// TwinCAT 3 PLC project DynTcComProxy
// ProgramVersion: 3.1.4024.0
// libraries:
//   Tc2_Standard, * (Beckhoff Automation GmbH)
//   Tc2_System, * (Beckhoff Automation GmbH)
//   Tc2_Utilities, * (Beckhoff Automation GmbH)
//   Tc3_Module, * (Beckhoff Automation GmbH)
//   TcComProxyApplication, * (YuYang_Beckhoffsh)
// project tree:
//   / PlcTask.TcTTO
//   POUs/ FB_DynProxyTcComConvertModule.TcPOU, MAIN.TcPOU
// real-time tasks:
//   TASK PlcTask: cycle T#10ms, priority 20, ADS port 350
//   TASK PlcTask1: cycle T#10ms, priority 21, ADS port 351
//   TASK PlcTask2: cycle T#10ms, priority 22, ADS port 352
//   TASK PlcTask3: cycle T#10ms, priority 23, ADS port 353
// variable links:
//   TcComPLCCaller/TcComPLCCaller Instance <-> TcComPLCProvider/TcComPLCProvider Instance
//     PlcTask Inputs/MAIN.fbProxyPLCCalculationTcComModule._objectId <-> PlcTask Outputs/MAIN.fbCalc.objID

CONFIGURATION DynTcComProxy
    RESOURCE PLC ON TwinCAT3
        TASK PlcTask(INTERVAL := T#10ms, PRIORITY := 20);
        PROGRAM MAIN WITH PlcTask : MAIN;
    END_RESOURCE
END_CONFIGURATION

// ---- POUs/MAIN.TcPOU
PROGRAM MAIN
VAR
	fbProxyConvert	: FB_DynProxyTcComConvertModule(	classID		:= STRING_TO_GUID('f229f89c-d59b-4036-b41f-784807c6fb38'),
														IID			:= TC_GLOBAL_IID_LIST.IID_IAnalogToPWM,
														sObjectName	:= 'DataConvertDrv:fbProxyConvert',
														eObjState   := TCOM_STATE.TCOM_STATE_OP);
	AnalogValue		: LREAL	:= 50;
	bPwmPos			: BOOL;
	bPwmNeg			: BOOL;
	TestCounter		: DINT;
	INITED			: BOOL	:= FALSE;
	binit			: BOOL;	
	
	hr				: HRESULT;

	bChange			: BOOL;
	bDelete			: BOOL;
	bExecute		: BOOL;
END_VAR



IF fbProxyConvert.ip <> 0 THEN

	fbProxyConvert.Cyclic();

	IF  binit THEN
		fbProxyConvert.ip.initParam(T#1S);
		binit:=FALSE;
		INITED:= TRUE;
	END_IF

	IF bExecute THEN
		hr := fbProxyConvert.ip.Convert(AnalogValue,ADR(bPwmPos),ADR(bPwmNeg),ADR(TestCounter));
	END_IF
	
	IF bChange THEN
		hr := fbProxyConvert.iTcComobject.TcSetObjState(TCOM_STATE.TCOM_STATE_PREOP,fbProxyConvert.iTComObjectServer,0);
	END_IF
END_IF


IF bDelete THEN
	fbProxyConvert.FB_exit(FALSE);
	bDelete:= FALSE;
END_IF

END_PROGRAM

// ---- POUs/FB_DynProxyTcComConvertModule.TcPOU
{attribute 'TcDependDnClassFactory ' := 'DataConvertDrv'}
FUNCTION_BLOCK FB_DynProxyTcComConvertModule EXTENDS FB_DynProxyTcComModule
VAR_INPUT
END_VAR
VAR_OUTPUT
END_VAR
VAR
	_iThisProvider		: IAnalogToPWM;
END_VAR

METHOD FB_exit : BOOL
VAR_INPUT
	bInCopyCode : BOOL; // if TRUE, the exit method is called for exiting an instance that is copied afterwards (online change).
END_VAR
IF NOT bInCopyCode THEN
	FW_SafeRelease(pipUnk:= ADR(_iThisProvider));
END_IF
END_METHOD

METHOD FB_init : BOOL
VAR_INPUT
	bInitRetains 	: BOOL; // if TRUE, the retain variables are initialized (warm start / cold start)
	bInCopyCode 	: BOOL;  // if TRUE, the instance afterwards gets moved into the copy code (online change)
	classID			: CLSID;
	IID				: IID;
	sObjectName		: STRING;
	eObjState		: TCOM_STATE;
END_VAR
ComQueryInterface(Super^._iProvider,TC_GLOBAL_IID_LIST.IID_IAnalogToPWM, ADR(_iThisProvider));
END_METHOD

PROPERTY ip : IAnalogToPWM
GET
ip	:= _iThisProvider;
END_GET
END_PROPERTY

END_FUNCTION_BLOCK
